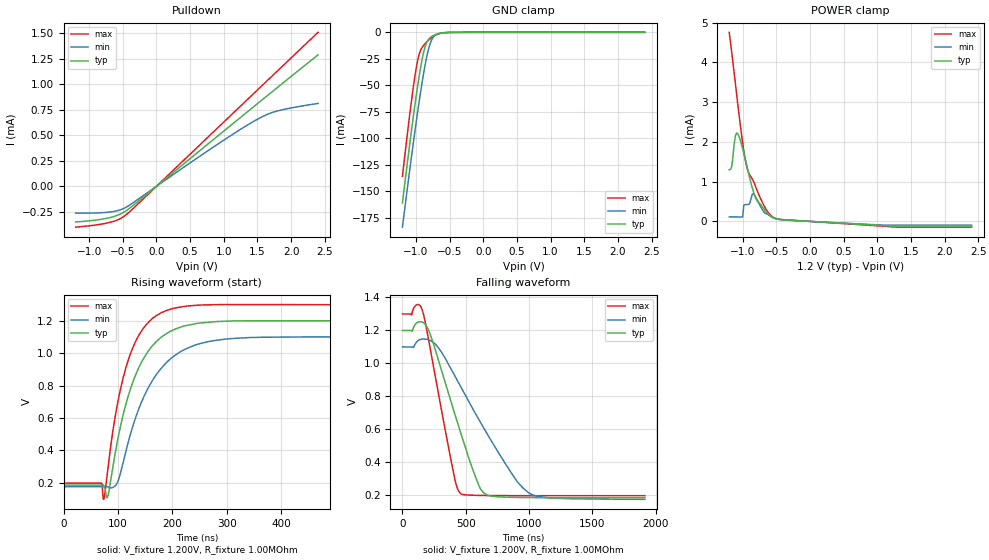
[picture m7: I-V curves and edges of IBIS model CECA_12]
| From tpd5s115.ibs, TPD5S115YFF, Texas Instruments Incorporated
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[Model]   CECA_12
Model_type   I/O_open_sink
Vinl = 800.000mV
Vinh = 2.000V
Vmeas = 1.500V
Cref = 15pF
Vref = 0V
Rref = 1000000
|   typ   min   max
|3-state
C_comp   1.2365pF   1.2156pF   1.2811pF
|pulldown
|C_comp   1.2367pF   1.2156pF   1.2806pF
[Voltage Range]   1.200V   1.10V   1.30V
|Junction temperature
[Temperature Range]   40.0   100.0   -40.0
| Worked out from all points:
|   slope of the pulldown table from 0 to 0.18 V, typ, clamps not added: 1.84 kohm
|   GND clamp passes 1 mA (typ) near -0.64 V on its own axis
|   POWER clamp passes 1 mA (typ) near -0.88 V on its own axis
|   falling waveform, V_fixture 1.200V, R_fixture 1.00MOhm: 20-80 % time 247ns typ, 419ns min, 160ns max; typ from 1.2 V to 0.185 V
|   rising waveform, V_fixture 1.200V, R_fixture 1.00MOhm: 20-80 % time 57.3ns typ, 69.6ns min, 47ns max; typ from 0.185 V to 1.2 V
|ambient temperature   25   85   -40|
[Pulldown]
|   Voltage   I(typ)   I(min)   I(max)
-1.2V     -349uA     -263uA     -400.3uA
-910.6mV  -331.8uA   -261.2uA   -379.7uA
-693.5mV  -307uA     -252.1uA   -353.9uA
-548.7mV  -275.6uA   -233.2uA   -320.6uA
-440.2mV  -234.7uA   -200.8uA   -273.3uA
898.5mV   486.5uA    408uA      565.7uA
1.26V     681.2uA    563uA      793.3uA
1.532V    826.8uA    668.3uA    963.8uA
1.676V    904.2uA    713uA      1.055mA
1.821V    981.4uA    742.6uA    1.146mA
2.4V      1.288mA    812.1uA    1.509mA
[GND Clamp]
|   Voltage   I(typ)   I(min)   I(max)
-1.2V     -160.9mA   -183.7mA   -135.7mA
-1.128V   -123.5mA   -147.5mA   -96.24mA
-1.055V   -87.61mA   -112.4mA   -59.51mA
-1.001V   -62.34mA   -87.12mA   -35.82mA
-964.8mV  -46.72mA   -70.98mA   -23.96mA
-910.6mV  -26.39mA   -48.32mA   -14.55mA
-856.3mV  -12.33mA   -28.52mA   -10.14mA
-820.1mV  -7.344mA   -17.81mA   -7.859mA
-783.9mV  -4.748mA   -9.908mA   -5.874mA
-711.6mV  -2.215mA   -2.556mA   -2.812mA
-476.4mV  -100.5uA   -89.62uA   -87.76uA
2.4V      0A         0A         0A
[POWER Clamp]
|   Voltage   I(typ)   I(min)   I(max)
-1.2V     1.301mA    114.1uA    4.759mA
-1.164V   1.376mA    113.7uA    4.266mA
-1.11V    2.148mA    112.9uA    3.485mA
-1.091V   2.222mA    112.6uA    3.222mA
-1.001V   1.832mA    112uA      1.979mA
-982.9mV  1.709mA    411.5uA    1.769mA
-946.7mV  1.452mA    423.1uA    1.426mA
-856.3mV  837.5uA    689.2uA    1.064mA
-802mV    565.3uA    599.6uA    849.4uA
-675.4mV  290.3uA    215uA      371.3uA
-566.8mV  117.9uA    106uA      127.7uA
2.4V      -117.9uA   -94.86uA   -144.7uA
[Ramp]
R_load = 1.00MOhm
|   typ   min   max
dV/dt_r   609.156mV/57.330ns  554.964mV/69.604ns  661.696mV/46.978ns
dV/dt_f   609.156mV/247.418ns 554.964mV/419.328ns 661.696mV/160.053ns
[Falling Waveform]
V_fixture = 1.200V
V_fixture_min = 1.100V
V_fixture_max = 1.300V
R_fixture = 1.00MOhm
|   Time   V(typ)   V(min)   V(max)
0s        1.2V       1.1V       1.3V
72ns      1.2V       1.1V       1.295V
118ns     1.248V     1.135V     1.357V
158ns     1.25V      1.148V     1.32V
223ns     1.169V     1.138V     1.075V
417ns     683.6mV    918.7mV    285.3mV
462ns     573.4mV    854.7mV    208.4mV
640ns     215.9mV    610.5mV    198.3mV
1.004us   185.7mV    211.7mV    197.2mV
1.914us   184.7mV    175mV      197.2mV
[Rising Waveform]
V_fixture = 1.200V
V_fixture_min = 1.100V
V_fixture_max = 1.300V
R_fixture = 1.00MOhm
|   Time   V(typ)   V(min)   V(max)
0s        184.7mV    175mV      197.2mV
70ns      184.7mV    175.1mV    196.5mV
74ns      182.1mV    175mV      96.62mV
82ns      123.2mV    173.1mV    302mV
100ns     473.1mV    208.2mV    702.3mV
125ns     798.8mV    523.3mV    1.015V
163ns     1.044V     829mV      1.214V
216ns     1.162V     1.011V     1.286V
380ns     1.201V     1.1V       1.3V
1.914us   1.2V       1.1V       1.3V
